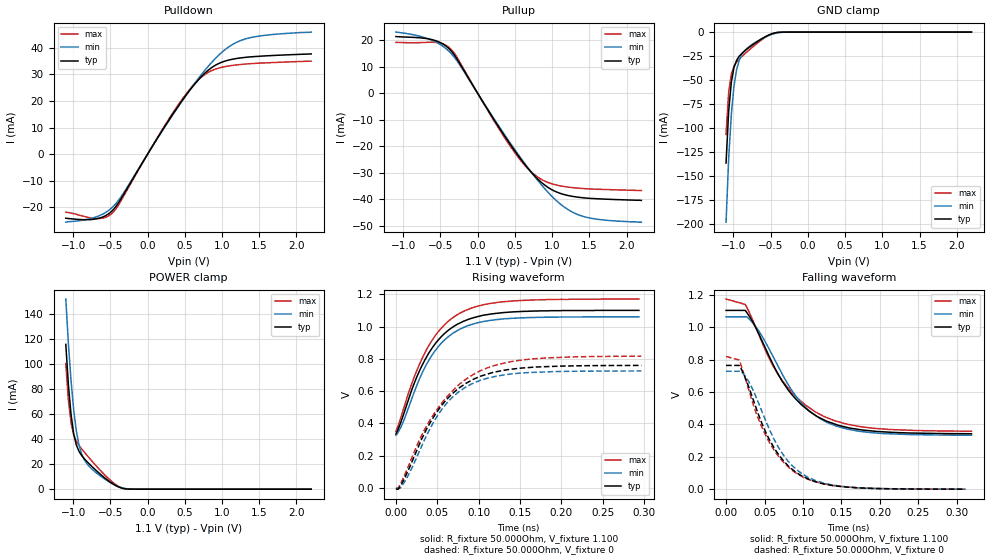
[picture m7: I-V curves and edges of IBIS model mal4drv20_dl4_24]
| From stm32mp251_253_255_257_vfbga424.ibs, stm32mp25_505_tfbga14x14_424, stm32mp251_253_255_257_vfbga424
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[Model] mal4drv20_dl4_24
Model_type   I/O
Polarity   Non-Inverting
Enable   Active-High
C_comp   1.837pF   1.837pF   1.849pF
C_comp_pullup   942.491fF   934.703fF   950.576fF
C_comp_pulldown 782.742fF   781.933fF   799.826fF
Vinh = 432.000mV
Vinl = 312.000mV
Vmeas = 372.000mV
Vref = 0.00V
Rref = 50Ohms
Cref = 0pF
[Model Spec]
Vinh   432.000mV   418.000mV   455.000mV
Vinl   312.000mV   298.000mV   335.000mV
Vmeas   372.000mV   358.000mV   395.000mV
Vref   0.00V   0.00V   0.00V
D_overshoot_ampl_h 0.3 NA   NA
D_overshoot_ampl_l 0.3 NA   NA
D_overshoot_area_l 100.000m NA   NA
D_overshoot_area_h 100.000m NA   NA
[Receiver Thresholds]
Vth = 372.000mV
Vth_min = 358.000mV
Vth_max = 395.000mV
Vinh_ac = 600.000mV
Vinh_dc = 600.000mV
Vinl_ac = -600.000mV
Vinl_dc = -600.000mV
Tslew_ac = 5.000ns
Threshold_sensitivity = 0.5
Reference_supply Pullup_ref
[Temperature Range]   25.000   125.000   -40.000
[Voltage Range]   1.100V   1.060V   1.170V
[GND Clamp Reference]   0.00V   0.00V   0.00V
[C Comp Corner]
| variable   typ   min   max
C_comp 1.849pF   1.837pF   1.837pF
C_comp_pullup 942.491fF   950.576fF   934.703fF
C_comp_pulldown 781.933fF   799.826fF   782.742fF
[Pulldown Reference]   0.00V   0.00V   0.00V
[POWER Clamp Reference]   1.100V   1.060V   1.170V
[Pullup Reference]   1.100V   1.060V   1.170V
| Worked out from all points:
|   slope of the pulldown table from 0 to 0.165 V, typ, clamps not added: 22 ohm
|   slope of the pullup table from 0 to 0.165 V, typ, clamps not added: 22 ohm
|   GND clamp passes 1 mA (typ) near -0.45 V on its own axis
|   POWER clamp passes 1 mA (typ) near -0.36 V on its own axis
|   rising waveform, R_fixture 50.000Ohm, V_fixture 1.100: 20-80 % time 45.5ps typ, 44.5ps min, 47.2ps max; typ from 0.336 V to 1.1 V
|   rising waveform, R_fixture 50.000Ohm, V_fixture 0: 20-80 % time 55.1ps typ, 51ps min, 62.1ps max; typ from -0.007 V to 0.759 V
|   falling waveform, R_fixture 50.000Ohm, V_fixture 1.100: 20-80 % time 61.3ps typ, 59.3ps min, 65.1ps max; typ from 1.1 V to 0.342 V
|   falling waveform, R_fixture 50.000Ohm, V_fixture 0: 20-80 % time 47.9ps typ, 48ps min, 48.4ps max; typ from 0.764 V to 0 V
[GND Clamp]
-1.099V   -136.3mA   -197.9mA   -106.5mA
-1.064V   -82.47mA   -132mA     -62.93mA
-1.028V   -52.05mA   -85.75mA   -43.61mA
-992.7mV  -36.88mA   -56.43mA   -35.5mA
-957.3mV  -29.36mA   -39.14mA   -31.26mA
-921.8mV  -25.1mA    -29.22mA   -28.2mA
-886.4mV  -22.16mA   -23.33mA   -25.51mA
-850.9mV  -19.73mA   -19.54mA   -22.95mA
-780mV    -15.43mA   -14.59mA   -18.04mA
-531.8mV  -3.288mA   -3.748mA   -3.604mA
-390mV    -251.1uA   -613.4uA   -163.8uA
2.198V    42.3nA     621.2nA    4.643nA
[Power Clamp]
-1.098V   115.5mA    151.6mA    100.1mA
-1.063V   83.06mA    116mA      70.82mA
-1.027V   59.24mA    86.19mA    52.7mA
-991.8mV  44.02mA    63.02mA    43.29mA
-956.4mV  35.26mA    46.38mA    38.3mA
-920.9mV  30.19mA    35.27mA    34.98mA
-885.5mV  26.87mA    28.15mA    32.19mA
-850mV    24.29mA    23.52mA    29.6mA
-672.7mV  13.97mA    12.28mA    17.45mA
-424.5mV  2.786mA    2.91mA     3.554mA
-282.7mV  160.9uA    380.1uA    143.1uA
2.199V    -14.13nA   -533.6nA   -2.884nA
[Pulldown]
-1.099V   -24.1mA    -25.6mA    -21.8mA
-673.6mV  -24.24mA   -23.43mA   -24.23mA
-567.3mV  -23.19mA   -22mA      -23.79mA
-460.9mV  -20.88mA   -19.65mA   -21.8mA
-319.1mV  -15.04mA   -14.44mA   -15.66mA
106.4mV   4.869mA    4.744mA    5.047mA
425.4mV   18.61mA    18.43mA    19.09mA
673.6mV   27.67mA    28.14mA    27.74mA
886.4mV   33.03mA    35.27mA    31.72mA
1.099V    35.44mA    40.51mA    33.21mA
1.312V    36.39mA    43.3mA     33.87mA
2.198V    37.7mA     45.9mA     34.98mA
[Pullup]
-1.098V   21.4mA     23.09mA    19.2mA
-601.8mV  20.16mA    19.86mA    19.26mA
-460mV    18.49mA    17.61mA    18.57mA
-353.6mV  15.91mA    14.92mA    16.51mA
249.1mV   -11.24mA   -10.86mA   -11.71mA
497.3mV   -21.66mA   -21.18mA   -22.32mA
710mV     -29.43mA   -29.4mA    -29.4mA
922.7mV   -35.07mA   -36.66mA   -33.39mA
1.135V    -37.98mA   -42.32mA   -35.04mA
1.384V    -39.31mA   -46.13mA   -35.84mA
1.667V    -39.86mA   -47.71mA   -36.24mA
2.199V    -40.4mA    -48.61mA   -36.67mA
[Ramp]
R_load=50.000Ohm
dV/dt_r   455.370mV/51.500ps  435.779mV/49.000ps  489.000mV/56.000ps
dV/dt_f   455.370mV/55.500ps  435.779mV/54.500ps  489.000mV/58.500ps
[Rising waveform]
R_fixture=50.000Ohm
V_fixture=1.100
V_fixture_min=1.060
V_fixture_max=1.170
0s        335.7mV    327.3mV    352.2mV
9ps       452.8mV    411.6mV    487.5mV
22ps      646.6mV    592.9mV    685.8mV
30ps      742.5mV    692.9mV    783.7mV
38ps      819.7mV    774.9mV    865.6mV
56ps      943.1mV    902.8mV    995.7mV
79ps      1.026V     987.6mV    1.087V
106ps     1.07V      1.031V     1.135V
140ps     1.09V      1.051V     1.158V
294ps     1.1V       1.06V      1.17V
[Rising waveform]
R_fixture=50.000Ohm
V_fixture=0
0s        -6.8mV     -675.8uV   -6.043mV
3ps       -6.8mV     -675.8uV   2.904mV
11ps      65.78mV    42.44mV    85.82mV
32ps      312.4mV    270.1mV    335.6mV
51ps      481.8mV    453.9mV    496.2mV
72ps      601.2mV    579.2mV    620.5mV
95ps      676.4mV    652.6mV    707.3mV
122ps     720.9mV    693mV      763.2mV
160ps     746.2mV    715mV      797.2mV
297ps     759.2mV    724.9mV    816.4mV
[Falling waveform]
R_fixture=50.000Ohm
V_fixture=1.100
V_fixture_min=1.060
V_fixture_max=1.170
0s        1.104V     1.064V     1.174V
25ps      1.104V     1.064V     1.141V
34ps      1.039V     1.031V     1.051V
58ps      800.4mV    847.9mV    788.8mV
72ps      674.3mV    719.3mV    677.9mV
97ps      525.5mV    537.9mV    545mV
126ps     431mV      425.8mV    451.7mV
156ps     382.9mV    372.3mV    402.7mV
186ps     361mV      350.2mV    379.5mV
319ps     342.4mV    333.3mV    358mV
[Falling waveform]
R_fixture=50.000Ohm
V_fixture=0
0s        764.2mV    728.1mV    819.6mV
17ps      764.2mV    728.1mV    797.5mV
25ps      687.7mV    697.8mV    683.1mV
40ps      488mV      558.4mV    459mV
57ps      300.5mV    362.3mV    283.2mV
79ps      152.2mV    182.1mV    145.4mV
100ps     78.51mV    91.49mV    74.8mV
126ps     33.96mV    38.53mV    33.09mV
154ps     14.06mV    15.39mV    14.16mV
311ps     153.5uV    183.3uV    178.6uV
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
